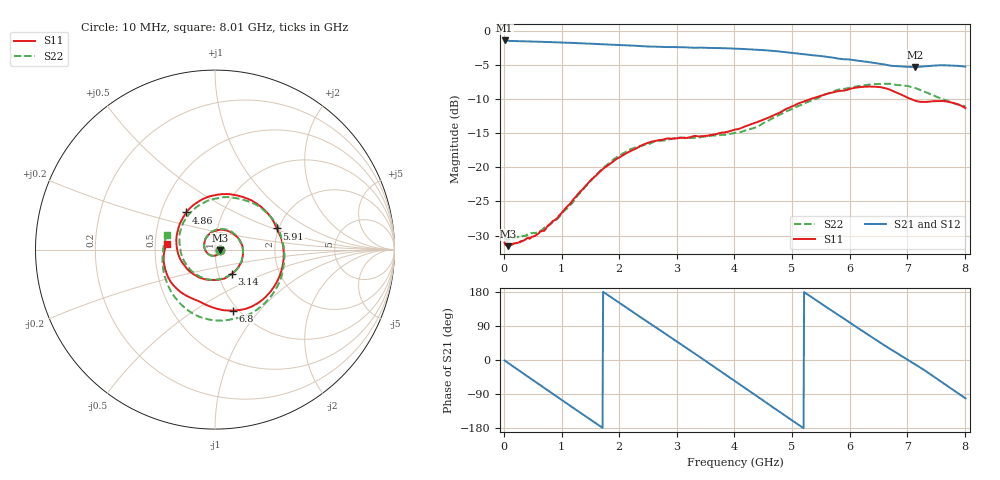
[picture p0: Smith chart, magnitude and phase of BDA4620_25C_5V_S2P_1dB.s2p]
!Agilent Technologies,E5071B,MY42404982,A.09.10
!Date: Wed May 06 08:58:17 2026
!Data & Calibration Information:
!Freq	S11:SOLT2(ON)	S21:SOLT2(ON)	S12:SOLT2(ON)	S22:SOLT2(ON)
# Hz S RI R 50
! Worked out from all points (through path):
!   801 points, 10 MHz to 8.01 GHz, reference 50 ohm
!   highest |S21| = -1.45 dB at 10 MHz (marker M1); lowest = -5.3 dB at 7.13 GHz (marker M2)
!   group delay of S21, straight-line fit = 285 ps
!   lowest |S11| = -31.6 dB at 70 MHz (marker M3), VSWR 1.05, Z = 52.7 - j0.463 ohm
!   |S11| at or under -10 dB: start of sweep to 5.328 GHz; 7.057 GHz to end of sweep
!   |S22| runs from -30.7 to -7.8 dB; largest |S21 - S12| = 0.0036
!   S11 on the Smith chart (normalised r, x): 10 MHz: 1.06, -0.00; 3.14 GHz: 1.16, -0.32; 4.86 GHz: 0.67, +0.30; 5.91 GHz: 1.96, +0.53; 6.8 GHz: 0.94, -0.73; 8.01 GHz: 0.58, +0.04
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1e7  0.028 -0.00199  0.8461 -0.0178  0.8471 -0.0181  0.0306 -0.00199
7e7  0.0261 -0.00439  0.8346 -0.1125  0.8354 -0.1138  0.0293 -0.00438
7.3e8  -0.00896 -0.0346  0.1852 -0.8038  0.1848 -0.8052  -0.00596 -0.0361
1.03e9  -0.0445 -0.0182  -0.2574 -0.7749  -0.2579 -0.7758  -0.0423 -0.0205
1.35e9  -0.0603 0.0314  -0.6333 -0.4997  -0.6339 -0.5003  -0.0606 0.0288
1.64e9  -0.035 0.0835  -0.7882 -0.1139  -0.789 -0.114  -0.0385 0.0827
1.93e9  0.0253 0.1102  -0.7299 0.2906  -0.7311 0.2915  0.0216 0.114
2.32e9  0.1161 0.0767  -0.3633 0.6814  -0.3647 0.6824  0.1153 0.0817
2.68e9  0.1569 -0.0166  0.1127 0.7527  0.1132 0.7536  0.1555 -0.00468
3.14e9  0.0951 -0.1333  0.6218 0.426  0.6233 0.425  0.1079 -0.1239
3.57e9  -0.0248 -0.1688  0.7351 -0.1273  0.7361 -0.1288  -0.0122 -0.1688
4.01e9  -0.1513 -0.1112  0.4151 -0.6092  0.4151 -0.6105  -0.1431 -0.1064
4.43e9  -0.2147 0.0301  -0.12 -0.7109  -0.1216 -0.7124  -0.1976 0.0368
4.86e9  -0.1602 0.2068  -0.5702 -0.4026  -0.5705 -0.4025  -0.1271 0.2162
5.35e9  0.0773 0.3093  -0.637 0.1727  -0.6373 0.1734  0.1136 0.2868
5.91e9  0.3444 0.1179  -0.1933 0.5849  -0.1933 0.5859  0.3654 0.0807
6.26e9  0.3716 -0.1126  0.1746 0.5663  0.1767 0.5667  0.3726 -0.1393
6.68e9  0.1753 -0.3287  0.475 0.2892  0.4769 0.2895  0.1967 -0.3577
6.8e9  0.099 -0.3394  0.5156 0.1904  0.5174 0.1905  0.1179 -0.3825
7.13e9  -0.0633 -0.3011  0.5307 -0.1028  0.5317 -0.1035  -0.1048 -0.3666
7.62e9  -0.2462 -0.1804  0.2766 -0.4829  0.2772 -0.4848  -0.2834 -0.1379
8.01e9  -0.269 0.0308  -0.1049 -0.5344  -0.1055 -0.5355  -0.2658 0.0831
